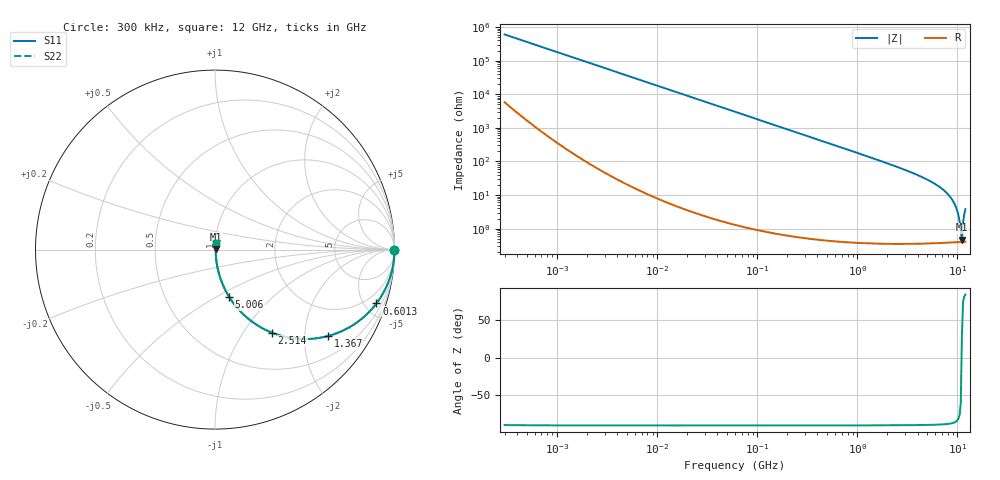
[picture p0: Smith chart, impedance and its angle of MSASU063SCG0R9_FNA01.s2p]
! MSASU063SCG0R9_FNA01  S-PARAMETER MODEL  ( Standard Model )
! Model Generated by TAIYO YUDEN Corporation (http://www.ty-top.com)
! Version 1.0
! TAIYO YUDEN Control No. 240819
! Copyright(c) 2024 TAIYO YUDEN CO.,LTD. All Rights Reserved.
! Product Description (link to TY-COMPAS)
! https://ds.yuden.co.jp/TYCOMPAS/or/detail?pn=MSASU063SCG0R9CFNA01&u=M
! Products Name : Multilayer Ceramic Capacitors
! Characteristics :
!  Capacitance : 0.9 [pF] , Rated Voltage : 50 [V] , TCC : CG / C0G
!  Case Size : 0.6 x 0.3 / 0.024 x 0.012 [mm/inch] , Thickness : 0.3 / 0.012 [mm/inch]
!  (Conditions: Temperature = 25 [degC] , DC Bias Voltage = 0 [V])
! External Node Assignments :
!  1  o---| |---o  2
! GND o---------o GND
! Frequency Range : 0.3MHz  -  12000MHz  [ 401 STEP ]
# MHZ S RI R 50
! Freq[MHz].  S11 Real  S11 Imag  S21 Real  S21 Imag  S12 Real  S12 Imag  S22 Real  S22 Imag
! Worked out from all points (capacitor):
!   401 points, 300 kHz to 12 GHz, reference 50 ohm
!   read as one part in series: C = 880 fF near 316.3 kHz
!   lowest |Z| = 467 mohm at 11.08 GHz (marker M1)
!   series resonance near 11.01 GHz, so ESL is about 240 pH
!   S11 on the Smith chart (normalised r, x): 300 kHz: open; 601.3 MHz: 1.01, -6.00; 1.367 GHz: 1.01, -2.61; 2.514 GHz: 1.01, -1.36; 5.006 GHz: 1.01, -0.57; 12 GHz: 1.01, +0.08
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0.3  1 -0.000166  1.62e-06 0.000166  1.62e-06 0.000166  1 -0.000166
1.769972  1 -0.000979  2.08e-06 0.000979  2.08e-06 0.000979  1 -0.000979
10.44266  1 -0.00577  3.58e-05 0.00577  3.58e-05 0.00577  1 -0.00577
60  0.9989 -0.0331  0.00111 0.0331  0.00111 0.0331  0.9989 -0.0331
164.1901  0.9918 -0.09  0.00823 0.09  0.00823 0.09  0.9918 -0.09
353.9943  0.9629 -0.1886  0.0371 0.1886  0.0371 0.1886  0.9629 -0.1886
601.3112  0.8996 -0.2998  0.1004 0.2998  0.1004 0.2998  0.8996 -0.2998
918.7169  0.7922 -0.4048  0.2078 0.4048  0.2078 0.4048  0.7922 -0.4048
1366.97  0.629 -0.4817  0.371 0.4817  0.371 0.4817  0.629 -0.4817
2088.533  0.4112 -0.4899  0.5888 0.4899  0.5888 0.4899  0.4112 -0.4899
2514.07  0.3184 -0.4633  0.6816 0.4633  0.6816 0.4633  0.3184 -0.4633
5006.236  0.0788 -0.2633  0.9212 0.2633  0.9212 0.2633  0.0788 -0.2633
6879.757  0.0286 -0.1554  0.9714 0.1554  0.9714 0.1554  0.0286 -0.1554
8503.825  0.0111 -0.0849  0.9889 0.0849  0.9889 0.0849  0.0111 -0.0849
9207.246  0.00736 -0.0588  0.9926 0.0588  0.9926 0.0588  0.00736 -0.0588
9708.23  0.00564 -0.0414  0.9944 0.0414  0.9944 0.0414  0.00564 -0.0414
9968.853  0.00501 -0.0328  0.995 0.0328  0.995 0.0328  0.00501 -0.0328
10511.28  0.00421 -0.0155  0.9958 0.0155  0.9958 0.0155  0.00421 -0.0155
10793.46  0.00404 -0.00691  0.996 0.00691  0.996 0.00691  0.00404 -0.00691
11083.22  0.00401 0.00235  0.996 -0.00235  0.996 -0.00235  0.00401 0.00235
11380.75  0.00424 0.0144  0.9958 -0.0144  0.9958 -0.0144  0.00424 0.0144
12000  0.00546 0.0373  0.9945 -0.0373  0.9945 -0.0373  0.00546 0.0373
